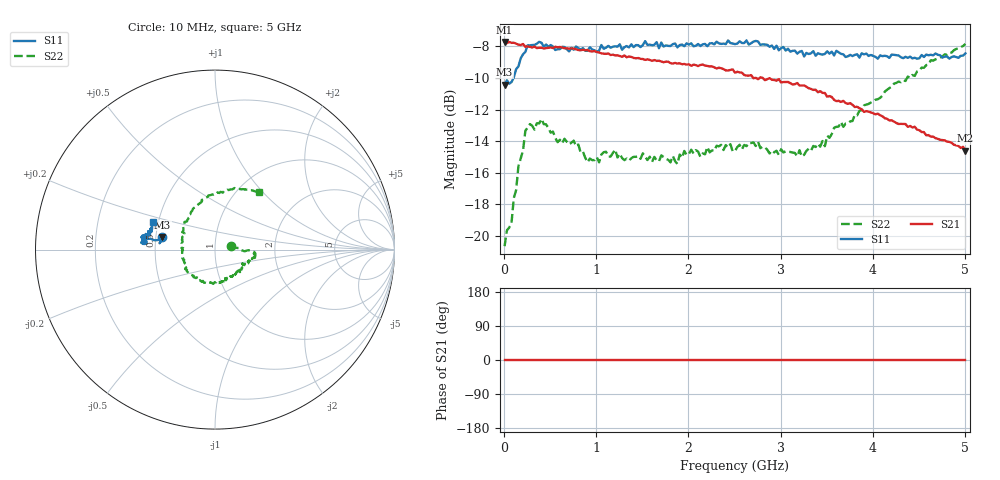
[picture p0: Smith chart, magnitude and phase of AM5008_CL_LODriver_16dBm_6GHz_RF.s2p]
!Keysight Technologies,N5245B,MY58422270,A.16.20.02
!Mixer S2P File: Scalar Mixer Measurement
!Calibration State: On
!Parameters: Stimulus Freq, S11, SC21, SC12, S22
# Hz  S  DB  R  50.0
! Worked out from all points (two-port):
!   201 points, 10 MHz to 5 GHz, reference 50 ohm
!   highest |S21| = -7.72 dB at 10 MHz (marker M1); lowest = -14.6 dB at 5 GHz (marker M2)
!   |S21| within 3 dB of the highest: start of sweep to 3.338 GHz
!   lowest |S11| = -10.4 dB at 10 MHz (marker M3), VSWR 1.86, Z = 27.1 + j4.22 ohm
!   |S11| at or under -10 dB: start of sweep to 106.6 MHz
!   |S22| runs from -20.6 to -7.9 dB; largest |S21 - S12| = 0.41
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1e7  -10.42 166.4  -7.72 0.0  -200.00 90.0  -20.64 10.9
3.495e7  -10.15 173.5  -7.80 0.0  -200.00 90.0  -19.64 4.5
8.485e7  -10.27 169.2  -7.78 0.0  -200.00 90.0  -19.18 5.5
1.597e8  -9.27 171.2  -7.89 0.0  -200.00 90.0  -15.58 -3.3
2.3455e8  -8.36 170.5  -8.04 0.0  -200.00 90.0  -13.35 -3.1
2.8445e8  -7.94 171.1  -8.04 0.0  -200.00 90.0  -12.92 -5.5
4.092e8  -7.78 171.5  -8.09 0.0  -200.00 90.0  -12.60 -8.5
5.8385e8  -8.18 172.8  -8.06 0.0  -200.00 90.0  -14.07 -16.5
8.583e8  -8.12 174.2  -8.22 0.0  -200.00 90.0  -14.66 -25.5
9.082e8  -8.28 174.8  -8.23 0.0  -200.00 90.0  -15.34 -26.8
1.2076e9  -8.00 174.2  -8.58 0.0  -200.00 90.0  -14.53 -41.9
1.68165e9  -8.12 173.6  -8.91 0.0  -200.00 90.0  -15.28 -59.9
2.2056e9  -7.99 172.0  -9.25 0.0  -200.00 90.0  -14.37 -92.8
2.505e9  -7.86 171.2  -9.67 0.0  -200.00 90.0  -14.62 -123.6
2.7545e9  -7.69 169.5  -10.09 0.0  -200.00 90.0  -14.04 -147.0
3.17865e9  -8.46 167.1  -10.32 0.0  -200.00 90.0  -14.96 -179.2
3.3533e9  -8.31 166.4  -10.76 0.0  -200.00 90.0  -14.30 163.3
3.47805e9  -8.48 166.0  -10.95 0.0  -200.00 90.0  -14.32 151.9
3.6527e9  -8.48 164.3  -11.52 0.0  -200.00 90.0  -12.79 137.7
4.17665e9  -8.73 161.0  -12.69 0.0  -200.00 90.0  -10.64 99.8
4.62575e9  -8.54 157.8  -13.72 0.0  -200.00 90.0  -8.88 72.5
5e9  -8.45 155.9  -14.61 0.0  -200.00 90.0  -7.85 52.3
